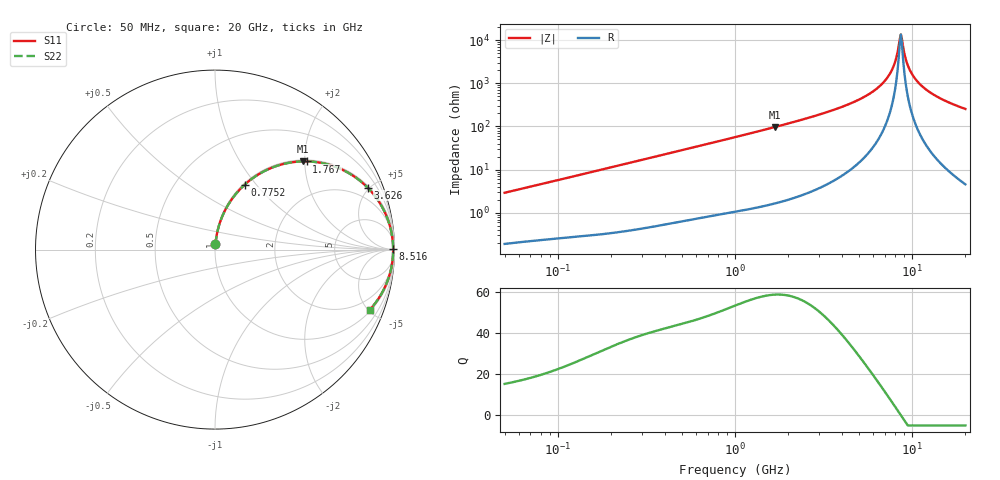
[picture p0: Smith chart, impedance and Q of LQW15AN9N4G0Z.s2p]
!Murata Part Number: LQW15AN9N4G0Z
!These Parameters are Measured in Series Mode Connection
!  o--[Z]--o
!Port1  Port2
!  o-------o
!Freq. Start=50[MHz] Stop=20[GHz], 401[Steps]
# Hz S RI R 50
!Freq.(Hz) S11(Real) S11(Imag) S21(Real) S21(Imag) S12(Real) S12(Imag) S22(Real) S22(Imag)
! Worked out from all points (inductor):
!   401 points, 50 MHz to 20 GHz, reference 50 ohm
!   read as one part in series: L = 9.2 nH near 51.52 MHz
!   highest Q = 58.8 at 1.689 GHz (marker M1), where L = 9.18 nH
!   self-resonance near 8.516 GHz
!   S11 on the Smith chart (normalised r, x): 50 MHz: 1.00, +0.06; 775.2 MHz: 1.02, +0.87; 1.767 GHz: 1.03, +2.05; 3.626 GHz: 1.11, +4.88; 8.516 GHz: open; 20 GHz: 1.09, -5.08
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5e7  0.00275 0.029  0.9973 -0.029  0.9973 -0.029  0.00275 0.029
1.364002e8  0.0088 0.0768  0.9912 -0.0768  0.9912 -0.0768  0.0088 0.0768
3.721004e8  0.0466 0.1992  0.9534 -0.1992  0.9534 -0.1992  0.0466 0.1992
7.751977e8  0.1649 0.3612  0.8351 -0.3612  0.8351 -0.3612  0.1649 0.3612
1e9  0.2458 0.4213  0.7542 -0.4213  0.7542 -0.4213  0.2458 0.4213
1.689197e9  0.4875 0.4914  0.5125 -0.4914  0.5125 -0.4914  0.4875 0.4914
1.766834e9  0.5113 0.4914  0.4887 -0.4914  0.4887 -0.4914  0.5113 0.4914
2.728004e9  0.7344 0.4324  0.2656 -0.4324  0.2656 -0.4324  0.7344 0.4324
3.626126e9  0.8504 0.3454  0.1496 -0.3454  0.1496 -0.3454  0.8504 0.3454
4.677679e9  0.924 0.2499  0.076 -0.2499  0.076 -0.2499  0.924 0.2499
5.769027e9  0.9636 0.1658  0.0364 -0.1658  0.0364 -0.1658  0.9636 0.1658
6.701223e9  0.9812 0.1045  0.0188 -0.1045  0.0188 -0.1045  0.9812 0.1045
7.442007e9  0.9887 0.0614  0.0113 -0.0614  0.0113 -0.0614  0.9887 0.0614
8.020766e9  0.9916 0.0306  0.00839 -0.0306  0.00839 -0.0306  0.9916 0.0306
8.516016e9  0.9926 0.00596  0.00742 -0.00596  0.00742 -0.00596  0.9926 0.00596
8.774992e9  0.9926 -0.00638  0.0074 0.00638  0.0074 0.00638  0.9926 -0.00638
9.316812e9  0.9917 -0.0311  0.00829 0.0311  0.00829 0.0311  0.9917 -0.0311
9.745021e9  0.9902 -0.0496  0.00976 0.0496  0.00976 0.0496  0.9902 -0.0496
1.034674e10  0.9872 -0.0742  0.0128 0.0742  0.0128 0.0742  0.9872 -0.0742
1.115139e10  0.9816 -0.1051  0.0184 0.1051  0.0184 0.1051  0.9816 -0.1051
1.417136e10  0.9495 -0.203  0.0505 0.203  0.0505 0.203  0.9495 -0.203
2e10  0.8614 -0.3366  0.1386 0.3366  0.1386 0.3366  0.8614 -0.3366
